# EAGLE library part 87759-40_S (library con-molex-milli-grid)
HEADER
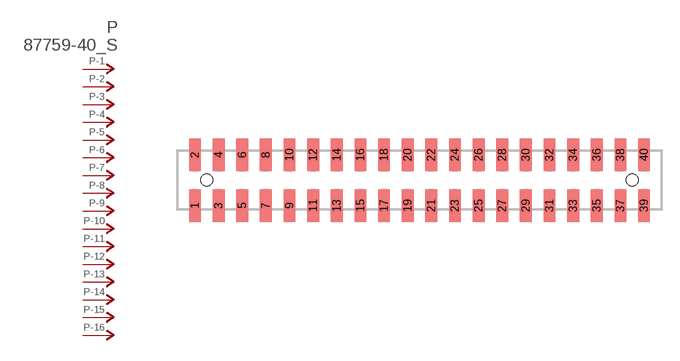
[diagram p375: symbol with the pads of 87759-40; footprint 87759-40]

Designator prefix P; gates -1=P-NV -2=P-N -3=P-N -4=P-N -5=P-N -6=P-N -7=P-N -8=P-N -9=P-N -10=P-N -11=P-N -12=P-N -13=P-N -14=P-N -15=P-N -16=P-N -17=P-N -18=P-N -19=P-N -20=P-N -21=P-N -22=P-N -23=P-N -24=P-N -25=P-N -26=P-N -27=P-N -28=P-N -29=P-N -30=P-N -31=P-N -32=P-N -33=P-N -34=P-N -35=P-N -36=P-N -37=P-N -38=P-N -39=P-N -40=P-N

## 87759-40_S  [87759-40]
1  -1:P  pas
2  -2:P  pas
3  -3:P  pas
4  -4:P  pas
5  -5:P  pas
6  -6:P  pas
7  -7:P  pas
8  -8:P  pas
9  -9:P  pas
10  -10:P  pas
11  -11:P  pas
12  -12:P  pas
13  -13:P  pas
14  -14:P  pas
15  -15:P  pas
16  -16:P  pas
17  -17:P  pas
18  -18:P  pas
19  -19:P  pas
20  -20:P  pas
21  -21:P  pas
22  -22:P  pas
23  -23:P  pas
24  -24:P  pas
25  -25:P  pas
26  -26:P  pas
27  -27:P  pas
28  -28:P  pas
29  -29:P  pas
30  -30:P  pas
31  -31:P  pas
32  -32:P  pas
33  -33:P  pas
34  -34:P  pas
35  -35:P  pas
36  -36:P  pas
37  -37:P  pas
38  -38:P  pas
39  -39:P  pas
40  -40:P  pas

## Footprint 87759-40 (pad centres in mm)
HEADER SMD Dual Row, Vertical
smd 1 x 2.75: 1 -19,-2.15; 2 -19,2.15; 3 -17,-2.15; 4 -17,2.15; 5 -15,-2.15; 6 -15,2.15; 7 -13,-2.15; 8 -13,2.15; 9 -11,-2.15; 10 -11,2.15; 11 -9,-2.15; 12 -9,2.15; 13 -7,-2.15; 14 -7,2.15; 15 -5,-2.15; 16 -5,2.15; 17 -3,-2.15; 18 -3,2.15; 19 -1,-2.15; 20 -1,2.15; 21 1,-2.15; 22 1,2.15; 23 3,-2.15; 24 3,2.15; 25 5,-2.15; 26 5,2.15; 27 7,-2.15; 28 7,2.15; 29 9,-2.15; 30 9,2.15; 31 11,-2.15; 32 11,2.15; 33 13,-2.15; 34 13,2.15; 35 15,-2.15; 36 15,2.15; 37 17,-2.15; 38 17,2.15; 39 19,-2.15; 40 19,2.15
hole 1 at -18,0
hole 1 at 18,0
